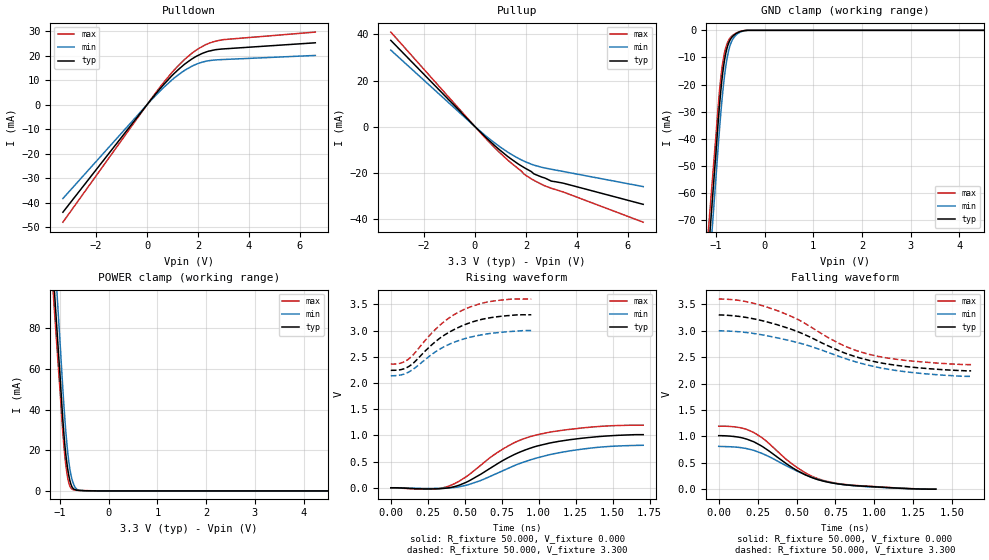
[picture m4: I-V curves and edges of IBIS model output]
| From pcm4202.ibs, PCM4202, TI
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[Model]   output
Model_type Output
Vref=0.000E+00
Rref=1.000E+06
Cref=1.500E-12
Vmeas=1.650E+00
C_comp   9.900E-13   9.880E-13   1.010E-12
[Voltage Range]   3.300E+00   3.000E+00   3.600E+00
[POWER Clamp Reference]   3.300E+00   3.000E+00   3.600E+00
[GND Clamp Reference]   0.000E+00   0.000E+00   0.000E+00
[Pullup Reference]   3.300E+00   3.000E+00   3.600E+00
[Pulldown Reference]   0.000E+00   0.000E+00   0.000E+00
[Temperature Range]   25   70   -10
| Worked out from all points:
|   slope of the pulldown table from 0 to 0.495 V, typ, clamps not added: 78.3 ohm
|   slope of the pullup table from 0 to 0.495 V, typ, clamps not added: 91.8 ohm
|   GND clamp passes 1 mA (typ) near -0.56 V on its own axis
|   POWER clamp passes 1 mA (typ) near -0.72 V on its own axis
|   rising waveform, R_fixture 50.000, V_fixture 0.000: 20-80 % time 437ps typ, 475ps min, 395ps max; typ from 0 V to 1.01 V
|   falling waveform, R_fixture 50.000, V_fixture 0.000: 20-80 % time 336ps typ, 365ps min, 317ps max; typ from 1.01 V to 0 V
|   rising waveform, R_fixture 50.000, V_fixture 3.300: 20-80 % time 301ps typ, 307ps min, 288ps max; typ from 2.24 V to 3.3 V
|   falling waveform, R_fixture 50.000, V_fixture 3.300: 20-80 % time 545ps typ, 586ps min, 502ps max; typ from 3.3 V to 2.24 V
[GND Clamp]
-3.3V     -594.8mA   -619.2mA   -559mA
-1.02V    -50.27mA   -59.71mA   -43.64mA
-940mV    -31.02mA   -39.98mA   -25.37mA
-900mV    -22.65mA   -30.92mA   -17.8mA
-860mV    -15.87mA   -23.04mA   -12.09mA
-800mV    -8.816mA   -13.78mA   -6.61mA
-760mV    -5.897mA   -9.384mA   -4.492mA
-700mV    -3.299mA   -5.147mA   -2.643mA
-640mV    -1.977mA   -2.907mA   -1.67mA
-540mV    -768uA     -1.05mA    -647.7uA
-340mV    0A         0A         0A
6.6V      0A         0A         0A
[Power Clamp]
-3.3V     891.7mA    975.1mA    843.7mA
-1.02V    63.8mA     80.91mA    55.99mA
-940mV    34.42mA    49.33mA    27.99mA
-900mV    22.41mA    35.18mA    16.83mA
-880mV    17.71mA    28.96mA    12.52mA
-840mV    10.45mA    18.55mA    6.172mA
-820mV    7.621mA    14.45mA    4.01mA
-780mV    3.552mA    8.365mA    1.558mA
-740mV    1.454mA    4.573mA    714.5uA
-660mV    404uA      925.2uA    318uA
-480mV    99.23uA    56.36uA    154uA
6.6V      0A         0A         0A
[Pullup]
-3.3V     37.41mA    33.19mA    41.01mA
380mV     -4.204mA   -3.617mA   -4.623mA
820mV     -8.717mA   -7.476mA   -9.668mA
1.28V     -12.92mA   -11.04mA   -14.44mA
1.82V     -17.05mA   -14.45mA   -19.31mA
1.92V     -17.72mA   -14.96mA   -20.56mA
2.2V      -19.44mA   -16.26mA   -22.59mA
2.3V      -20.41mA   -16.65mA   -23.22mA
2.74V     -22.3mA    -17.96mA   -25.71mA
3V        -23.67mA   -18.51mA   -26.77mA
3.46V     -24.54mA   -19.47mA   -28.35mA
6.6V      -33.73mA   -26.03mA   -41.47mA
[Pulldown]
-3.3V     -43.9mA    -38.31mA   -47.97mA
0V        0A         0A         0A
480mV     6.141mA    5.273mA    6.774mA
1.06V     12.71mA    10.84mA    14.11mA
1.46V     16.43mA    13.92mA    18.35mA
1.76V     18.67mA    15.71mA    21.01mA
2.28V     21.38mA    17.67mA    24.42mA
2.68V     22.44mA    18.27mA    25.9mA
2.98V     22.76mA    18.44mA    26.55mA
6.6V      25.27mA    20.11mA    29.64mA
[Rising Waveform]
R_fixture = 50.000
V_fixture = 0.000
V_fixture_min = 0.000
V_fixture_max = 0.000
|  time   V(typ)   V(min)   V(max)
0s        0V         0V         0V
262.5ps   -21.75mV   -13.38mV   -26.33mV
390ps     -1.601mV   -5.427mV   29.79mV
527.5ps   128.6mV    61.72mV    245.9mV
675ps     376.9mV    220.7mV    583.2mV
762.5ps   527.7mV    330.8mV    746.5mV
870ps     676.7mV    461.1mV    902.8mV
992.5ps   797.9mV    572.2mV    1.013V
1.343ns   959.6mV    753.7mV    1.154V
1.707ns   1.013V     810.4mV    1.193V
[Falling Waveform]
R_fixture = 50.000
V_fixture = 0.000
V_fixture_min = 0.000
V_fixture_max = 0.000
|  time   V(typ)   V(min)   V(max)
0s        1.013V     810.4mV    1.193V
130ps     983.9mV    790.8mV    1.168V
220ps     903.5mV    738.9mV    1.081V
292.5ps   784.4mV    658.2mV    942.5mV
422.5ps   507.3mV    460.4mV    593.5mV
497.5ps   363.5mV    350.2mV    421.5mV
590ps     229.3mV    234.1mV    257.8mV
667.5ps   155.8mV    160.3mV    170.3mV
895ps     63.2mV     59.31mV    67.64mV
1.395ns   0V         0V         0V
[Rising Waveform]
R_fixture = 50.000
V_fixture = 3.300
V_fixture_min = 3.000
V_fixture_max = 3.600
|  time   V(typ)   V(min)   V(max)
0s        2.241V     2.136V     2.358V
65ps      2.252V     2.151V     2.377V
117.5ps   2.307V     2.202V     2.449V
332.5ps   2.856V     2.647V     3.104V
410ps     2.991V     2.756V     3.27V
487.5ps   3.097V     2.834V     3.391V
597.5ps   3.2V       2.909V     3.505V
677.5ps   3.246V     2.946V     3.556V
812.5ps   3.289V     2.982V     3.598V
950ps     3.3V       3V         3.6V
[Falling Waveform]
R_fixture = 50.000
V_fixture = 3.300
V_fixture_min = 3.000
V_fixture_max = 3.600
|  time   V(typ)   V(min)   V(max)
0s        3.3V       3V         3.6V
172.5ps   3.254V     2.968V     3.554V
385ps     3.105V     2.86V      3.371V
507.5ps   2.983V     2.775V     3.216V
770ps     2.626V     2.518V     2.765V
882.5ps   2.506V     2.409V     2.626V
965ps     2.44V      2.345V     2.554V
1.08ns    2.372V     2.275V     2.485V
1.267ns   2.303V     2.201V     2.419V
1.622ns   2.241V     2.136V     2.358V
[Ramp]
dV/dt_r   6.1203E-01/4.3463E-10   4.8646E-01/4.7340E-10   7.1644E-01/3.9500E-10
dV/dt_f   6.3545E-01/5.4359E-10   5.1832E-01/5.8531E-10   7.4517E-01/5.0150E-10
R_load = 50
